FUNCTION_BLOCK FB_SortingModule EXTENDS FB_Module
// Module to select via sensor, cylinder and axis
VAR_INPUT
		(* Variables to enable / disable diagnosis and temperature mode *)
	bCylinderDiag				: BOOL;
	bCylinderTemp				: BOOL;
	bCylinderRecord				: BOOL;
		(* Buttons *)
	bButtonCylToWorkIn			: BOOL;
	bButtonCylToBaseIn			: BOOL;
		(* Timer values *)
	tiTimeOutCylinder			: TIME;
	tiRecordIntervall			: TIME;
	tiSensorDelay				: TIME;
	tiMoveAxis					: TIME;					// Time to move axis
END_VAR
VAR_OUTPUT
	bToWork						: BOOL;
	bAtBase						: BOOL;
	bAtWork						: BOOL;
	bCylError					: BOOL;
	sCylErrorMsg				: STRING;
	lrTemps						: ARRAY[1..100] OF LREAL;
	bSelected					: BOOL;
	bButtonCylToWorkOut			: BOOL;
	bButtonCylToBaseOut			: BOOL;
END_VAR
VAR
(* ================= Function block and interface instances ===================== *)
	
	fbSensorDelay				: FB_SignalHandlingDelay;
		(* Instances of cylinder function blocks *)
	fbCylinder					: FB_Cylinder;					// Without diagnosis and temperature mode
	fbCylinderDiag				: FB_CylinderDiag;				// With diagnosis of states
	fbCylinderTemp				: FB_CylinderTemp;				// With temperature mode
	fbCylinderTempDiag			: FB_CylinderTempDiag;			// With diagnosis of temperature
	fbCylinderTempRecord		: FB_CylinderTempRecord;		// With record of temperatures
		(* Interface instance of ICylinder for cylinder *)
	iCyl						: ICylinder;
	
		(***** Manual cylinder control *****)
	fbButtonCylToWork			: FB_SignalHandlingIntern;		// To move manually cylinder to work position
	fbButtonCylToBase			: FB_SignalHandlingIntern;		// To move manually cylinder to base position

(* ========================== COMMON VARIABLES =============================== *)
	tonAxis						: TON;							// Timer to move axis in (SEMI-) AUTOMATIC mode	
	rtrigCylAtWork				: R_TRIG;						// To diagnose rising edge of being in work position
END_VAR

// =========================================================
;
// =========================================================

METHOD PUBLIC M_Automatic
VAR_INPUT
END_VAR
// =========================================================
		// Selecting boxes via cylinder and axis

tonAxis( PT := tiMoveAxis );
rtrigCylAtWork( CLK := iCyl.P_AtWorkPos );			(***** Accessing property of FB via interface *****)

IF rtrigCylAtWork.Q THEN
	tonAxis( IN := TRUE );
END_IF

IF bSelected THEN
	bSelected := FALSE;
END_IF

IF tonAxis.Q THEN
	tonAxis( IN := FALSE );
	bSelected := TRUE;
	bHalt := TRUE;
	M_Stop();
ELSIF tonAxis.IN AND NOT bHalt THEN
	fbAxis.M_MoveFw();
END_IF

IF NOT bHaltDone THEN
	IF bHalt THEN
		M_Stop();
	END_IF
ELSE
	bHalt := FALSE;
	M_Stop();
END_IF

// =========================================================

CASE iState OF
	0:	// Detecting a box
		iCyl.M_MoveToBase();						(***** Calling method of FB via interface *****)
		IF fbSensorDelay.bOut THEN
			iState := 1;
		END_IF
			
	1: 	// Moving cylinder to work position
		iCyl.M_MoveToWork();						(***** Calling method of FB via interface *****)
		IF iCyl.P_AtWorkPos THEN					(***** Accessing property of FB via interface *****)
			iState := 2;
		END_IF
	
	2:	// Moving cylinder back to base position
		iCyl.M_MoveToBase();						(***** Calling method of FB via interface *****)	
		IF iCyl.P_AtBasePos THEN					(***** Accessing property of FB via interface *****)
			iState := 0;
		END_IF
END_CASE

// =========================================================
END_METHOD

METHOD PUBLIC M_CylinderOptions
VAR_INPUT
END_VAR
// =========================================================
			// Selecting cylinder

// Checking variables to enable / disable diagnosis and temperature mode
IF bCylinderDiag THEN
	IF bCylinderTemp THEN
		
	(* ============== FB with diagnosis and temperature mode ============== *)
		bCylError := fbCylinderTempDiag.bError;		// Assigning global output variable to output variable of selected FB
		sCylErrorMsg := fbCylinderTempDiag.sErrorMsg;
		iCyl := fbCylinderTempDiag;					// Assigning desired FB instance to interface instance
	
	ELSE
	
	(* ============== FB with diagnosis and without temperature mode ============== *)
		fbCylinderDiag.tiTimeOut := tiTimeOutCylinder;			// Setting special data for selected FB
		bCylError := fbCylinderDiag.bError;			// Assigning global output variable to output variable of selected FB
		sCylErrorMsg := fbCylinderDiag.sErrorMsg;
		iCyl := fbCylinderDiag;						// Assigning desired FB instance to interface instance
	END_IF
ELSE
	bCylError := FALSE;
	sCylErrorMsg := '';
	
	IF bCylinderTemp THEN
		IF bCylinderRecord THEN
			fbCylinderTempRecord.tiIntervalTime := tiRecordIntervall;	// Time of record interval
			fbCylinderTempRecord.bRecordStart := bComprAirEnabled;		// Recording if compressed air is set
			fbCylinderTempRecord.M_Record();							// Calling method of function block FB_CylinderTempRecord
			lrTemps := fbCylinderTempRecord.lrTemps;					// Saving output variable
			iCyl := fbCylinderTempRecord;
		ELSE
			(* ============== FB without diagnosis and with temperature mode ============== *)
			iCyl := fbCylinderTemp; 						// Assigning desired FB instance to interface instance
		END_IF
	ELSE
	
	(* ============== FB without diagnosis and temperature mode ============== *)
		iCyl := fbCylinder;							// Assigning desired FB instance to interface instance						
	END_IF	
END_IF
									
// =========================================================
END_METHOD

METHOD PUBLIC M_Enable
VAR_INPUT
END_VAR
// =========================================================
		// Calling method M_Enable of base class FB_Module via 'SUPER^.'
		
SUPER^.M_Enable();

// =========================================================
		// Sensor control
		
fbSensorDelay.bEnable := bSensorEnable;

// =========================================================
		// Cylinder control
		
fbButtonCylToWork.bEnable := bManualCylinderEnable
								AND NOT iCyl.P_AtWorkPos;		(*** Accessing property of FB via interface instance ***)
fbButtonCylToBase.bInput := NOT fbButtonCylToWork.bInput;
fbButtonCylToBase.bEnable := bManualCylinderEnable
								AND NOT iCyl.P_AtBasePos;		(*** Accessing property of FB via interface instance ***)

// =========================================================
END_METHOD

METHOD PUBLIC M_Maintenance
VAR_INPUT
END_VAR
// =========================================================
		// Calling own method M_Manual of this class FB_SortingModule via 'THIS^.'
		
THIS^.M_Manual();

// =========================================================
END_METHOD

METHOD PUBLIC M_Manual
VAR_INPUT
END_VAR
// =========================================================
		// Calling method M_Manual of base class FB_Module via 'SUPER^.'
		
SUPER^.M_Manual();

// =========================================================
	// Manual cylinder control
	
IF fbButtonCylToWork.bOut THEN
	iCyl.M_MoveToWork();				(**** Calling method of FB via interface instance ****)
ELSIF fbButtonCylToBase.bOut THEN
	iCyl.M_MoveToBase();				(**** Calling method of FB via interface instance ****)
END_IF

// =========================================================
END_METHOD

METHOD PUBLIC M_Reset
VAR_INPUT
END_VAR
// =========================================================
		// Resetting cylinder and axis
		
rtrigResetStart( CLK := bReset );

IF rtrigResetStart.Q THEN
	bSelected := FALSE;
	tonAxis( IN := FALSE );
	iCyl.M_Reset();						(**** Calling method of FB via interface ****)
END_IF

// =========================================================
		// Calling method of base class
		
SUPER^.M_Reset();						// Calling action M_Reset of base class FB_Module via 'SUPER^.'

// =========================================================
END_METHOD

METHOD PUBLIC M_Semiautomatic
VAR_INPUT
END_VAR
// =========================================================
		// Calling own method M_Automatic of this class FB_SortingModule via 'THIS^.'
		
THIS^.M_Automatic();				

// =========================================================
END_METHOD

METHOD PUBLIC M_SetOutput
VAR_INPUT
END_VAR
// =========================================================
		// Calling method M_SetOutput of base class FB_Module via 'SUPER^.'
		
SUPER^.M_SetOutput();

// =========================================================
		// Sensor
		
fbSensorDelay.M_SetOutput();

// =========================================================
		// Cylinder buttons
		
fbButtonCylToWork.M_SetOutput();
fbButtonCylToBase.M_SetOutput();

// =========================================================
		// Output variables for cylinder
		
bToWork := iCyl.P_ToWork;			// Assigning global output variable to property of selected FB
									// Accessing property of selected FB via interface instance
bAtBase := iCyl.P_AtBasePos;
bAtWork := iCyl.P_AtWorkPos;

// =========================================================
		// Buttons
		
fbButtonCylToWork.bInput := bButtonCylToWorkIn;
fbButtonCylToBase.bInput := bButtonCylToBaseIn;
bButtonCylToWorkOut := fbButtonCylToWork.bOut;
bButtonCylToBaseOut := fbButtonCylToBase.bOut;

// =========================================================
END_METHOD

METHOD PUBLIC M_Starting
VAR_INPUT
END_VAR
// =========================================================
		// Setting time to delay sensor
		
fbSensorDelay.tiDelay := tiSensorDelay;

// =========================================================
		// Calling method M_Starting of base class FB_Module via 'SUPER^.'
		
SUPER^.M_Starting();

// =========================================================
END_METHOD

END_FUNCTION_BLOCK
